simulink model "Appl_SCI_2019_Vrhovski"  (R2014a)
settings: Solver=ode45  StartTime=0.0  StopTime=1000  MaxStep=0.01  RelTol=1e-3
undefined symbols (not defined in the file): deg, H, kg, m, M, mm, N, rad, s, X, Y, Z
libraries: sm_lib x389, nesl_utility x69, simulink x7
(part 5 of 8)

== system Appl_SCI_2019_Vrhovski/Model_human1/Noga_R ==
  koljeno : Subsystem
  natkoljenica : Subsystem
  potkoljenica : Subsystem
  skocni_zglob_R : Subsystem
  skocni_zglob_R Joint : sm_lib/Joints/Universal Joint  SenseConstraintForce=off  SenseConstraintForceX=off  SenseConstraintForceY=off  SenseConstraintForceZ=off  SenseConstraintTorque=off  SenseConstraintTorqueX=off  SenseConstraintTorqueY=off  SenseConstraintTorqueZ=off  SenseTotalForce=off  SenseTotalForceX=off  SenseTotalForceY=off  SenseTotalForceZ=off  SenseTotalTorque=off  SenseTotalTorqueX=off  SenseTotalTorqueY=off  SenseTotalTorqueZ=off  CompositeWrenchDir=FollowerOnBase  CompositeWrenchFrame=BaseFrame  RxEquilibriumPosition=0  RxEquilibriumPositionUnits=deg  RxSpringStiffness=0  RxSpringStiffnessUnits=N*m/deg  RxDampingCoefficient=0  RxDampingCoefficientUnits=N*m/(deg/s)  RxTorqueActuationMode=ComputedTorque  RxMotionActuationMode=InputMotion  RxSensePosition=off  RxSenseVelocity=off  RxSenseAcceleration=off  RxSenseTorqueForce=off  RxPositionTargetValue=-0.08  RxPositionTargetValueUnits=rad  RxPositionTargetSpecify=on  RxPositionTargetPriority=High  RxVelocityTargetValue=0  RxVelocityTargetValueUnits=deg/s  RxVelocityTargetSpecify=off  RxVelocityTargetPriority=High  RyEquilibriumPosition=0  RyEquilibriumPositionUnits=deg  RySpringStiffness=0  RySpringStiffnessUnits=N*m/deg  RyDampingCoefficient=0  RyDampingCoefficientUnits=N*m/(deg/s)  RyTorqueActuationMode=ComputedTorque  RyMotionActuationMode=InputMotion  RySensePosition=off  RySenseVelocity=off  RySenseAcceleration=off  RySenseTorqueForce=off  RyPositionTargetValue=0  RyPositionTargetValueUnits=deg  RyPositionTargetSpecify=off  RyPositionTargetPriority=High  RyVelocityTargetValue=0  RyVelocityTargetValueUnits=deg/s  RyVelocityTargetSpecify=off  RyVelocityTargetPriority=High  BlockFunction=simmechanics.library.joints.universal_joint
  B : PMIOPort  Port=1  Side=Left
  F : PMIOPort  Port=2  Side=Right
  Nagib_skocnog : PMIOPort  Port=3  Side=Left
  RL1 : PMIOPort  Port=4  Side=Right
  RL2 : PMIOPort  Port=5  Side=Right
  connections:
  F/RConn1 -- natkoljenica/RConn1
  B/RConn1 -- skocni_zglob_R/LConn1
  koljeno/LConn1 -- potkoljenica/RConn1
  potkoljenica/LConn1 -- skocni_zglob_R Joint/RConn1
  skocni_zglob_R Joint/LConn1 -- RL1/RConn1 -- skocni_zglob_R/RConn1
  koljeno/RConn1 -- RL2/RConn1 -- natkoljenica/LConn1
  Nagib_skocnog/RConn1 -- skocni_zglob_R Joint/LConn3

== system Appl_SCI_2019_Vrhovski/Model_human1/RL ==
  L1 : Subsystem
  L2 : Subsystem
  L3 : Subsystem
  B : PMIOPort  Port=1  Side=Left
  FL1 : PMIOPort  Port=2  Side=Left
  FL2 : PMIOPort  Port=3  Side=Left
  FL3 : PMIOPort  Port=4  Side=Left
  Lxyz1 : Outport
  Lxyz2 : Outport  Port=2
  Lxyz3 : Outport  Port=3
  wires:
  L2/1(xyz) -> Lxyz2/1
  L3/1(xyz) -> Lxyz3/1
  L1/1(xyz) -> Lxyz1/1
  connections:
  FL2/RConn1 -- L2/LConn2
  L1/LConn2 -- FL1/RConn1
  L3/LConn2 -- FL3/RConn1
  B/RConn1 -- L1/LConn1 -- L3/LConn1 -- L2/LConn1

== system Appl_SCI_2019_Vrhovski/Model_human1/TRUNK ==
  T1 : Subsystem
  T2 : Subsystem
  T3 : Subsystem
  B : PMIOPort  Port=1  Side=Left
  FT1 : PMIOPort  Port=2  Side=Left
  FT2 : PMIOPort  Port=3  Side=Left
  FT3 : PMIOPort  Port=4  Side=Left
  Txyz1 : Outport
  Txyz2 : Outport  Port=2
  Txyz3 : Outport  Port=3
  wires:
  T1/1(xyz) -> Txyz1/1
  T3/1(xyz) -> Txyz3/1
  T2/1(xyz) -> Txyz2/1
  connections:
  T2/LConn1 -- T3/LConn1 -- T1/LConn1 -- B/RConn1
  T3/LConn2 -- FT3/RConn1
  T1/LConn2 -- FT1/RConn1
  FT2/RConn1 -- T2/LConn2

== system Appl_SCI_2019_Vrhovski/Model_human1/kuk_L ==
  Revolute Joint1 : sm_lib/Joints/Revolute Joint  SenseConstraintForce=off  SenseConstraintForceX=off  SenseConstraintForceY=off  SenseConstraintForceZ=off  SenseConstraintTorque=off  SenseConstraintTorqueX=off  SenseConstraintTorqueY=off  SenseConstraintTorqueZ=off  SenseTotalForce=off  SenseTotalForceX=off  SenseTotalForceY=off  SenseTotalForceZ=off  SenseTotalTorque=off  SenseTotalTorqueX=off  SenseTotalTorqueY=off  SenseTotalTorqueZ=off  CompositeWrenchDir=FollowerOnBase  CompositeWrenchFrame=BaseFrame  EquilibriumPosition=0  EquilibriumPositionUnits=deg  SpringStiffness=0  SpringStiffnessUnits=N*m/deg  DampingCoefficient=0  DampingCoefficientUnits=N*m/(deg/s)  TorqueActuationMode=NoTorque  MotionActuationMode=ComputedMotion  SensePosition=off  SenseVelocity=off  SenseAcceleration=off  SenseTorqueForce=off  PositionTargetValue=0  PositionTargetValueUnits=deg  PositionTargetSpecify=off  PositionTargetPriority=High  VelocityTargetValue=0  VelocityTargetValueUnits=deg/s  VelocityTargetSpecify=off  VelocityTargetPriority=High  BlockFunction=simmechanics.library.joints.revolute_joint
  Transform : sm_lib/Frames and Transforms/Rigid Transform  TranslationMethod=None  TranslationLengthUnit=mm  TranslationStandardAxis=+Z  TranslationStandardOffset=0  TranslationCartesianOffset=[-2.2026824808563106e-13 549.99999999999943 3.4106051316484809e-13]  TranslationROffset=0  TranslationROffsetUnits=m  TranslationZOffset=0  TranslationZOffsetUnits=m  TranslationThetaOffset=0  TranslationThetaOffsetUnits=deg  RotationMethod=StandardAxis  RotationAngleUnits=rad  RotationStandardAxis=+X  RotationAngle=pi/2  RotationArbitraryAxis=[0.57735026918962595 -0.57735026918962618 0.57735026918962518]  FollAlignAxisA=+X  BaseAlignAxisA=+Y  FollAlignAxisB=+Y  BaseAlignAxisB=+Z  BlockFunction=simmechanics.library.frames_transforms.rigid_transform
  Transform1 : sm_lib/Frames and Transforms/Rigid Transform  TranslationMethod=None  TranslationLengthUnit=mm  TranslationStandardAxis=+Z  TranslationStandardOffset=0  TranslationCartesianOffset=[-2.2026824808563106e-13 549.99999999999943 3.4106051316484809e-13]  TranslationROffset=0  TranslationROffsetUnits=m  TranslationZOffset=0  TranslationZOffsetUnits=m  TranslationThetaOffset=0  TranslationThetaOffsetUnits=deg  RotationMethod=StandardAxis  RotationAngleUnits=rad  RotationStandardAxis=-X  RotationAngle=pi/2  RotationArbitraryAxis=[0.57735026918962595 -0.57735026918962618 0.57735026918962518]  FollAlignAxisA=+X  BaseAlignAxisA=+Y  FollAlignAxisB=+Y  BaseAlignAxisB=+Z  BlockFunction=simmechanics.library.frames_transforms.rigid_transform
  kuk : Subsystem
  kuk_in : PMIOPort  Port=1  Side=Left
  kuk_out : PMIOPort  Port=2  Side=Right
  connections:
  Transform1/RConn1 -- kuk_out/RConn1
  Transform1/LConn1 -- Revolute Joint1/RConn1
  Transform/RConn1 -- Revolute Joint1/LConn1
  Transform/LConn1 -- kuk/RConn1
  kuk_in/RConn1 -- kuk/LConn1

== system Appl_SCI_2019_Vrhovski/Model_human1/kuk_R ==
  Revolute Joint1 : sm_lib/Joints/Revolute Joint  SenseConstraintForce=off  SenseConstraintForceX=off  SenseConstraintForceY=off  SenseConstraintForceZ=off  SenseConstraintTorque=off  SenseConstraintTorqueX=off  SenseConstraintTorqueY=off  SenseConstraintTorqueZ=off  SenseTotalForce=off  SenseTotalForceX=off  SenseTotalForceY=off  SenseTotalForceZ=off  SenseTotalTorque=off  SenseTotalTorqueX=off  SenseTotalTorqueY=off  SenseTotalTorqueZ=off  CompositeWrenchDir=FollowerOnBase  CompositeWrenchFrame=BaseFrame  EquilibriumPosition=0  EquilibriumPositionUnits=deg  SpringStiffness=0  SpringStiffnessUnits=N*m/deg  DampingCoefficient=0  DampingCoefficientUnits=N*m/(deg/s)  TorqueActuationMode=NoTorque  MotionActuationMode=ComputedMotion  SensePosition=off  SenseVelocity=off  SenseAcceleration=off  SenseTorqueForce=off  PositionTargetValue=0  PositionTargetValueUnits=deg  PositionTargetSpecify=off  PositionTargetPriority=High  VelocityTargetValue=0  VelocityTargetValueUnits=deg/s  VelocityTargetSpecify=off  VelocityTargetPriority=High  BlockFunction=simmechanics.library.joints.revolute_joint
  Transform : sm_lib/Frames and Transforms/Rigid Transform  TranslationMethod=None  TranslationLengthUnit=mm  TranslationStandardAxis=+Z  TranslationStandardOffset=0  TranslationCartesianOffset=[-2.2026824808563106e-13 549.99999999999943 3.4106051316484809e-13]  TranslationROffset=0  TranslationROffsetUnits=m  TranslationZOffset=0  TranslationZOffsetUnits=m  TranslationThetaOffset=0  TranslationThetaOffsetUnits=deg  RotationMethod=StandardAxis  RotationAngleUnits=rad  RotationStandardAxis=+X  RotationAngle=pi/2  RotationArbitraryAxis=[0.57735026918962595 -0.57735026918962618 0.57735026918962518]  FollAlignAxisA=+X  BaseAlignAxisA=+Y  FollAlignAxisB=+Y  BaseAlignAxisB=+Z  BlockFunction=simmechanics.library.frames_transforms.rigid_transform
  Transform1 : sm_lib/Frames and Transforms/Rigid Transform  TranslationMethod=None  TranslationLengthUnit=mm  TranslationStandardAxis=+Z  TranslationStandardOffset=0  TranslationCartesianOffset=[-2.2026824808563106e-13 549.99999999999943 3.4106051316484809e-13]  TranslationROffset=0  TranslationROffsetUnits=m  TranslationZOffset=0  TranslationZOffsetUnits=m  TranslationThetaOffset=0  TranslationThetaOffsetUnits=deg  RotationMethod=StandardAxis  RotationAngleUnits=rad  RotationStandardAxis=-X  RotationAngle=pi/2  RotationArbitraryAxis=[0.57735026918962595 -0.57735026918962618 0.57735026918962518]  FollAlignAxisA=+X  BaseAlignAxisA=+Y  FollAlignAxisB=+Y  BaseAlignAxisB=+Z  BlockFunction=simmechanics.library.frames_transforms.rigid_transform
  kuk : Subsystem
  kuk_in : PMIOPort  Port=1  Side=Left
  kuk_out : PMIOPort  Port=2  Side=Right
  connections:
  kuk_in/RConn1 -- kuk/LConn1
  Transform/LConn1 -- kuk/RConn1
  Transform/RConn1 -- Revolute Joint1/LConn1
  Transform1/LConn1 -- Revolute Joint1/RConn1
  Transform1/RConn1 -- kuk_out/RConn1

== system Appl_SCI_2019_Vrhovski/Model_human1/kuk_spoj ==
  ReferenceFrame : sm_lib/Frames and Transforms/Reference Frame  BlockFunction=simmechanics.library.frames_transforms.reference_frame
  Solid : sm_lib/Body Elements/Solid  InertiaType=Custom  Mass=0.1117*M  MassUnits=kg  CenterOfMass=[0 0 0]  CenterOfMassUnits=mm  MomentsOfInertia=[9638.0119049841542 90952.357607822152 82817.580647608978]  MomentsOfInertiaUnits=kg*mm^2  ProductsOfInertia=[101.02531458452592 0 0]  ProductsOfInertiaUnits=kg*mm^2  DensityBased=on  Density=1000  DensityUnits=kg/(m^3)  GraphicType=FromGeometry  MarkerShape=Sphere  MarkerSize=10  MarkerSizeUnits=m  GraphicVisPropType=SimpleVisualProperties  GraphicDiffuseColor=[0.792156862745098 0.81960784313725488 0.93333333333333335]  GraphicSpecularColor=[0.5 0.5 0.5 1.0]  GraphicAmbientColor=[0.15 0.15 0.15 1.0]  GraphicEmissiveColor=[0.0 0.0 0.0 1.0]  GraphicShininess=75  GraphicOpacity=1  GeometryShape=Ellipsoid  RectangleSize=[1 1]  RectangleSizeUnits=m  BrickDimensions=[330 50 50]  BrickDimensionUnits=mm  CylinderRadius=1  CylinderRadiusUnits=m  CylinderLength=1  CylinderLengthUnits=m  SphereRadius=1  SphereRadiusUnits=m  EllipsoidRadii=[175 50 0.05*H*5]  EllipsoidRadiiUnits=mm  ExtrusionCrossSection=[1 1; -1 1; -1 -1; 1 -1]  ExtrusionCrossSectionUnits=m  ExtrusionLength=1  ExtrusionLengthUnits=m  PolygonNumSides=3  PolygonOuterRadius=1  PolygonOuterRadiusUnits=m  ExtGeomFileType=STL  ExtGeomFileName=Spojnica_Default_sldprt.STL  ExtGeomFileUnits=mm  RevolutionCrossSection=[1 1; 1 -1; 2 -1; 2 1]  RevolutionCrossSectionUnits=m  RevolutionExtent=Full  RevolutionAngle=180  RevolutionAngleUnits=deg  BlockFunction=simmechanics.library.body_elements.solid
  Transform1 : sm_lib/Frames and Transforms/Rigid Transform  TranslationMethod=Cartesian  TranslationLengthUnit=mm  TranslationStandardAxis=+Z  TranslationStandardOffset=0  TranslationCartesianOffset=[132.5 0 0]  TranslationROffset=0  TranslationROffsetUnits=m  TranslationZOffset=0  TranslationZOffsetUnits=m  TranslationThetaOffset=0  TranslationThetaOffsetUnits=deg  RotationMethod=None  RotationAngleUnits=rad  RotationStandardAxis=+X  RotationAngle=pi  RotationArbitraryAxis=[0 0 0]  FollAlignAxisA=+X  BaseAlignAxisA=+Y  FollAlignAxisB=+Y  BaseAlignAxisB=+Z  BlockFunction=simmechanics.library.frames_transforms.rigid_transform
  Transform2 : sm_lib/Frames and Transforms/Rigid Transform  TranslationMethod=Cartesian  TranslationLengthUnit=mm  TranslationStandardAxis=+Z  TranslationStandardOffset=0  TranslationCartesianOffset=[-132.5 0 0]  TranslationROffset=0  TranslationROffsetUnits=m  TranslationZOffset=0  TranslationZOffsetUnits=m  TranslationThetaOffset=0  TranslationThetaOffsetUnits=deg  RotationMethod=None  RotationAngleUnits=rad  RotationStandardAxis=+X  RotationAngle=pi  RotationArbitraryAxis=[0 0 0]  FollAlignAxisA=+X  BaseAlignAxisA=+Y  FollAlignAxisB=+Y  BaseAlignAxisB=+Z  BlockFunction=simmechanics.library.frames_transforms.rigid_transform
  Transform3 : sm_lib/Frames and Transforms/Rigid Transform  TranslationMethod=None  TranslationLengthUnit=mm  TranslationStandardAxis=+Z  TranslationStandardOffset=0  TranslationCartesianOffset=[0 -0 -0]  TranslationROffset=0  TranslationROffsetUnits=m  TranslationZOffset=0  TranslationZOffsetUnits=m  TranslationThetaOffset=0  TranslationThetaOffsetUnits=deg  RotationMethod=None  RotationAngleUnits=rad  RotationStandardAxis=+X  RotationAngle=pi  RotationArbitraryAxis=[0 0 0]  FollAlignAxisA=+X  BaseAlignAxisA=+Y  FollAlignAxisB=+Y  BaseAlignAxisB=+Z  BlockFunction=simmechanics.library.frames_transforms.rigid_transform
  BL : PMIOPort  Port=1  Side=Right
  BR : PMIOPort  Port=2  Side=Right
  F : PMIOPort  Port=3  Side=Left
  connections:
  ReferenceFrame/RConn1 -- Transform3/LConn1 -- Solid/RConn1 -- Transform1/LConn1 -- Transform2/LConn1
  Transform1/RConn1 -- BR/RConn1
  Transform2/RConn1 -- BL/RConn1
  Transform3/RConn1 -- F/RConn1

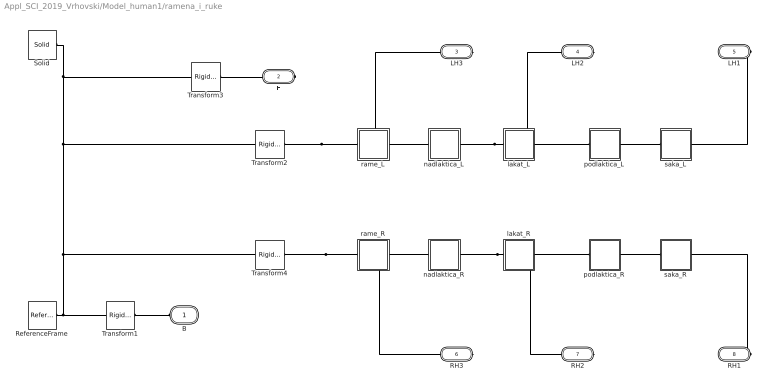
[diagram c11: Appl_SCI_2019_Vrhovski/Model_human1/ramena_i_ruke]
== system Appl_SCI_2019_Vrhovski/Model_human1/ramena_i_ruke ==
  ReferenceFrame : sm_lib/Frames and Transforms/Reference Frame  BlockFunction=simmechanics.library.frames_transforms.reference_frame
  Solid : sm_lib/Body Elements/Solid  InertiaType=Custom  Mass=0  MassUnits=kg  CenterOfMass=[0 0 0]  CenterOfMassUnits=mm  MomentsOfInertia=[9638.0119049841542 90952.357607822152 82817.580647608978]  MomentsOfInertiaUnits=kg*mm^2  ProductsOfInertia=[101.02531458452592 0 0]  ProductsOfInertiaUnits=kg*mm^2  DensityBased=on  Density=1000  DensityUnits=kg/(m^3)  GraphicType=FromGeometry  MarkerShape=Sphere  MarkerSize=10  MarkerSizeUnits=m  GraphicVisPropType=SimpleVisualProperties  GraphicDiffuseColor=[0.792156862745098 0.81960784313725488 0.93333333333333335]  GraphicSpecularColor=[0.5 0.5 0.5 1.0]  GraphicAmbientColor=[0.15 0.15 0.15 1.0]  GraphicEmissiveColor=[0.0 0.0 0.0 1.0]  GraphicShininess=75  GraphicOpacity=1  GeometryShape=Ellipsoid  RectangleSize=[1 1]  RectangleSizeUnits=m  BrickDimensions=[460 50 50]  BrickDimensionUnits=mm  CylinderRadius=1  CylinderRadiusUnits=m  CylinderLength=1  CylinderLengthUnits=m  SphereRadius=1  SphereRadiusUnits=m  EllipsoidRadii=[230 25 25]  EllipsoidRadiiUnits=mm  ExtrusionCrossSection=[1 1; -1 1; -1 -1; 1 -1]  ExtrusionCrossSectionUnits=m  ExtrusionLength=1  ExtrusionLengthUnits=m  PolygonNumSides=3  PolygonOuterRadius=1  PolygonOuterRadiusUnits=m  ExtGeomFileType=STL  ExtGeomFileName=Spojnica_Default_sldprt.STL  ExtGeomFileUnits=mm  RevolutionCrossSection=[1 1; 1 -1; 2 -1; 2 1]  RevolutionCrossSectionUnits=m  RevolutionExtent=Full  RevolutionAngle=180  RevolutionAngleUnits=deg  BlockFunction=simmechanics.library.body_elements.solid
  Transform1 : sm_lib/Frames and Transforms/Rigid Transform  TranslationMethod=StandardAxis  TranslationLengthUnit=mm  TranslationStandardAxis=+Z  TranslationStandardOffset=225  TranslationCartesianOffset=[150 0 0]  TranslationROffset=0  TranslationROffsetUnits=m  TranslationZOffset=0  TranslationZOffsetUnits=m  TranslationThetaOffset=0  TranslationThetaOffsetUnits=deg  RotationMethod=None  RotationAngleUnits=rad  RotationStandardAxis=+X  RotationAngle=pi  RotationArbitraryAxis=[0 0 0]  FollAlignAxisA=+X  BaseAlignAxisA=+Y  FollAlignAxisB=+Y  BaseAlignAxisB=+Z  BlockFunction=simmechanics.library.frames_transforms.rigid_transform
  Transform2 : sm_lib/Frames and Transforms/Rigid Transform  TranslationMethod=Cartesian  TranslationLengthUnit=mm  TranslationStandardAxis=+Z  TranslationStandardOffset=150  TranslationCartesianOffset=[200 0 -0]  TranslationROffset=0  TranslationROffsetUnits=m  TranslationZOffset=0  TranslationZOffsetUnits=m  TranslationThetaOffset=0  TranslationThetaOffsetUnits=deg  RotationMethod=StandardAxis  RotationAngleUnits=rad  RotationStandardAxis=+X  RotationAngle=pi  RotationArbitraryAxis=[0 0 0]  FollAlignAxisA=+X  BaseAlignAxisA=+Y  FollAlignAxisB=+Y  BaseAlignAxisB=+Z  BlockFunction=simmechanics.library.frames_transforms.rigid_transform
  Transform3 : sm_lib/Frames and Transforms/Rigid Transform  TranslationMethod=StandardAxis  TranslationLengthUnit=mm  TranslationStandardAxis=+Z  TranslationStandardOffset=150  TranslationCartesianOffset=[0 -0 -0]  TranslationROffset=0  TranslationROffsetUnits=m  TranslationZOffset=0  TranslationZOffsetUnits=m  TranslationThetaOffset=0  TranslationThetaOffsetUnits=deg  RotationMethod=None  RotationAngleUnits=rad  RotationStandardAxis=+X  RotationAngle=pi  RotationArbitraryAxis=[0 0 0]  FollAlignAxisA=+X  BaseAlignAxisA=+Y  FollAlignAxisB=+Y  BaseAlignAxisB=+Z  BlockFunction=simmechanics.library.frames_transforms.rigid_transform
  Transform4 : sm_lib/Frames and Transforms/Rigid Transform  TranslationMethod=Cartesian  TranslationLengthUnit=mm  TranslationStandardAxis=+Z  TranslationStandardOffset=150  TranslationCartesianOffset=[-200 0 -0]  TranslationROffset=0  TranslationROffsetUnits=m  TranslationZOffset=0  TranslationZOffsetUnits=m  TranslationThetaOffset=0  TranslationThetaOffsetUnits=deg  RotationMethod=StandardAxis  RotationAngleUnits=rad  RotationStandardAxis=+X  RotationAngle=pi  RotationArbitraryAxis=[0 0 0]  FollAlignAxisA=+X  BaseAlignAxisA=+Y  FollAlignAxisB=+Y  BaseAlignAxisB=+Z  BlockFunction=simmechanics.library.frames_transforms.rigid_transform
  lakat_L : Subsystem
  lakat_R : Subsystem
  nadlaktica_L : Subsystem
  nadlaktica_R : Subsystem
  podlaktica_L : Subsystem
  podlaktica_R : Subsystem
  rame_L : Subsystem
  rame_R : Subsystem
  saka_L : Subsystem
  saka_R : Subsystem
  B : PMIOPort  Port=1  Side=Left
  F : PMIOPort  Port=2  Side=Right
  LH3 : PMIOPort  Port=3  Side=Right
  LH2 : PMIOPort  Port=4  Side=Right
  LH1 : PMIOPort  Port=5  Side=Right
  RH3 : PMIOPort  Port=6  Side=Right
  RH2 : PMIOPort  Port=7  Side=Right
  RH1 : PMIOPort  Port=8  Side=Right
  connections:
  ReferenceFrame/RConn1 -- Transform1/LConn1 -- Transform4/LConn1 -- Transform2/LConn1 -- Transform3/LConn1 -- Solid/RConn1
  Transform1/RConn1 -- B/RConn1
  Transform3/RConn1 -- F/RConn1
  Transform2/RConn1 -- LH3/RConn1 -- rame_L/LConn1
  lakat_L/LConn1 -- LH2/RConn1 -- nadlaktica_L/RConn1
  saka_L/LConn1 -- podlaktica_L/RConn1
  saka_R/LConn1 -- podlaktica_R/RConn1
  lakat_R/LConn1 -- RH2/RConn1 -- nadlaktica_R/RConn1
  Transform4/RConn1 -- RH3/RConn1 -- rame_R/LConn1
  rame_L/RConn1 -- nadlaktica_L/LConn1
  nadlaktica_R/LConn1 -- rame_R/RConn1
  lakat_L/RConn1 -- podlaktica_L/LConn1
  lakat_R/RConn1 -- podlaktica_R/LConn1
  LH1/RConn1 -- saka_L/RConn1
  RH1/RConn1 -- saka_R/RConn1

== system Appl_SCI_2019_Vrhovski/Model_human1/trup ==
  ReferenceFrame : sm_lib/Frames and Transforms/Reference Frame  BlockFunction=simmechanics.library.frames_transforms.reference_frame
  Solid : sm_lib/Body Elements/Solid  InertiaType=Custom  Mass=0.1633*M  MassUnits=kg  CenterOfMass=[0 0 0]  CenterOfMassUnits=mm  MomentsOfInertia=[2897.1863857204326 1.8962829928219973 2897.1862300567827]  MomentsOfInertiaUnits=kg*mm^2  ProductsOfInertia=[0 0 -0.00027890183916846033]  ProductsOfInertiaUnits=kg*mm^2  DensityBased=on  Density=1000  DensityUnits=kg/(m^3)  GraphicType=FromGeometry  MarkerShape=Sphere  MarkerSize=10  MarkerSizeUnits=m  GraphicVisPropType=SimpleVisualProperties  GraphicDiffuseColor=[0.792156862745098 0.81960784313725488 0.93333333333333335]  GraphicSpecularColor=[0.5 0.5 0.5 1.0]  GraphicAmbientColor=[0.15 0.15 0.15 1.0]  GraphicEmissiveColor=[0.0 0.0 0.0 1.0]  GraphicShininess=75  GraphicOpacity=1  GeometryShape=Ellipsoid  RectangleSize=[1 1]  RectangleSizeUnits=m  BrickDimensions=[1 1 1]  BrickDimensionUnits=m  CylinderRadius=2.5  CylinderRadiusUnits=cm  CylinderLength=22  CylinderLengthUnits=cm  SphereRadius=5  SphereRadiusUnits=cm  EllipsoidRadii=[150 50 0.107*H*5]  EllipsoidRadiiUnits=mm  ExtrusionCrossSection=[1 1; -1 1; -1 -1; 1 -1]  ExtrusionCrossSectionUnits=m  ExtrusionLength=1  ExtrusionLengthUnits=m  PolygonNumSides=3  PolygonOuterRadius=1  PolygonOuterRadiusUnits=m  ExtGeomFileType=STL  ExtGeomFileName=Pod_Default_sldprt.STL  ExtGeomFileUnits=mm  RevolutionCrossSection=[1 1; 1 -1; 2 -1; 2 1]  RevolutionCrossSectionUnits=m  RevolutionExtent=Full  RevolutionAngle=180  RevolutionAngleUnits=deg  BlockFunction=simmechanics.library.body_elements.solid
  Transform1 : sm_lib/Frames and Transforms/Rigid Transform  TranslationMethod=StandardAxis  TranslationLengthUnit=mm  TranslationStandardAxis=+Z  TranslationStandardOffset=0.107*H*5 +10  TranslationCartesianOffset=[1.3358203432289883e-12 650.00000000000045 -1.0913936421275139e-11]  TranslationROffset=0  TranslationROffsetUnits=m  TranslationZOffset=0  TranslationZOffsetUnits=m  TranslationThetaOffset=0  TranslationThetaOffsetUnits=deg  RotationMethod=None  RotationAngleUnits=rad  RotationStandardAxis=+Z  RotationAngle=0  RotationArbitraryAxis=[0 0 0]  FollAlignAxisA=+X  BaseAlignAxisA=+Y  FollAlignAxisB=+Y  BaseAlignAxisB=+Z  BlockFunction=simmechanics.library.frames_transforms.rigid_transform
  Transform3 : sm_lib/Frames and Transforms/Rigid Transform  TranslationMethod=StandardAxis  TranslationLengthUnit=mm  TranslationStandardAxis=-Z  TranslationStandardOffset=0.107*H*5 +10  TranslationCartesianOffset=[-2.2026824808563106e-13 549.99999999999943 3.4106051316484809e-13]  TranslationROffset=0  TranslationROffsetUnits=m  TranslationZOffset=0  TranslationZOffsetUnits=m  TranslationThetaOffset=0  TranslationThetaOffsetUnits=deg  RotationMethod=None  RotationAngleUnits=rad  RotationStandardAxis=+Z  RotationAngle=2.0943951023931962  RotationArbitraryAxis=[0.57735026918962595 -0.57735026918962618 0.57735026918962518]  FollAlignAxisA=+X  BaseAlignAxisA=+Y  FollAlignAxisB=+Y  BaseAlignAxisB=+Z  BlockFunction=simmechanics.library.frames_transforms.rigid_transform
  F : PMIOPort  Port=1  Side=Right
  B : PMIOPort  Port=2  Side=Left
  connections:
  Transform1/LConn1 -- ReferenceFrame/RConn1 -- Solid/RConn1 -- Transform3/LConn1
  Transform1/RConn1 -- F/RConn1
  Transform3/RConn1 -- B/RConn1

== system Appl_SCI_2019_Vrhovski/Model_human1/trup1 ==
  ReferenceFrame : sm_lib/Frames and Transforms/Reference Frame  BlockFunction=simmechanics.library.frames_transforms.reference_frame
  Solid : sm_lib/Body Elements/Solid  InertiaType=Custom  Mass=0.17275*M  MassUnits=kg  CenterOfMass=[0 0 0]  CenterOfMassUnits=mm  MomentsOfInertia=[2897.1863857204326 1.8962829928219973 2897.1862300567827]  MomentsOfInertiaUnits=kg*mm^2  ProductsOfInertia=[0 0 -0.00027890183916846033]  ProductsOfInertiaUnits=kg*mm^2  DensityBased=on  Density=1000  DensityUnits=kg/(m^3)  GraphicType=FromGeometry  MarkerShape=Sphere  MarkerSize=10  MarkerSizeUnits=m  GraphicVisPropType=SimpleVisualProperties  GraphicDiffuseColor=[0.792156862745098 0.81960784313725488 0.93333333333333335]  GraphicSpecularColor=[0.5 0.5 0.5 1.0]  GraphicAmbientColor=[0.15 0.15 0.15 1.0]  GraphicEmissiveColor=[0.0 0.0 0.0 1.0]  GraphicShininess=75  GraphicOpacity=1  GeometryShape=Ellipsoid  RectangleSize=[1 1]  RectangleSizeUnits=m  BrickDimensions=[1 1 1]  BrickDimensionUnits=m  CylinderRadius=2.5  CylinderRadiusUnits=cm  CylinderLength=22  CylinderLengthUnits=cm  SphereRadius=5  SphereRadiusUnits=cm  EllipsoidRadii=[150 50 0.181*H*5]  EllipsoidRadiiUnits=mm  ExtrusionCrossSection=[1 1; -1 1; -1 -1; 1 -1]  ExtrusionCrossSectionUnits=m  ExtrusionLength=1  ExtrusionLengthUnits=m  PolygonNumSides=3  PolygonOuterRadius=1  PolygonOuterRadiusUnits=m  ExtGeomFileType=STL  ExtGeomFileName=Pod_Default_sldprt.STL  ExtGeomFileUnits=mm  RevolutionCrossSection=[1 1; 1 -1; 2 -1; 2 1]  RevolutionCrossSectionUnits=m  RevolutionExtent=Full  RevolutionAngle=180  RevolutionAngleUnits=deg  BlockFunction=simmechanics.library.body_elements.solid
  Transform1 : sm_lib/Frames and Transforms/Rigid Transform  TranslationMethod=StandardAxis  TranslationLengthUnit=mm  TranslationStandardAxis=+Z  TranslationStandardOffset=0.181*H*5+10  TranslationCartesianOffset=[1.3358203432289883e-12 650.00000000000045 -1.0913936421275139e-11]  TranslationROffset=0  TranslationROffsetUnits=m  TranslationZOffset=0  TranslationZOffsetUnits=m  TranslationThetaOffset=0  TranslationThetaOffsetUnits=deg  RotationMethod=None  RotationAngleUnits=rad  RotationStandardAxis=+Z  RotationAngle=0  RotationArbitraryAxis=[0 0 0]  FollAlignAxisA=+X  BaseAlignAxisA=+Y  FollAlignAxisB=+Y  BaseAlignAxisB=+Z  BlockFunction=simmechanics.library.frames_transforms.rigid_transform
  Transform3 : sm_lib/Frames and Transforms/Rigid Transform  TranslationMethod=StandardAxis  TranslationLengthUnit=mm  TranslationStandardAxis=-Z  TranslationStandardOffset=0.181*H*5+10  TranslationCartesianOffset=[-2.2026824808563106e-13 549.99999999999943 3.4106051316484809e-13]  TranslationROffset=0  TranslationROffsetUnits=m  TranslationZOffset=0  TranslationZOffsetUnits=m  TranslationThetaOffset=0  TranslationThetaOffsetUnits=deg  RotationMethod=None  RotationAngleUnits=rad  RotationStandardAxis=+Z  RotationAngle=2.0943951023931962  RotationArbitraryAxis=[0.57735026918962595 -0.57735026918962618 0.57735026918962518]  FollAlignAxisA=+X  BaseAlignAxisA=+Y  FollAlignAxisB=+Y  BaseAlignAxisB=+Z  BlockFunction=simmechanics.library.frames_transforms.rigid_transform
  F : PMIOPort  Port=1  Side=Right
  B : PMIOPort  Port=2  Side=Left
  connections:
  Transform3/RConn1 -- B/RConn1
  Transform1/RConn1 -- F/RConn1
  Transform3/LConn1 -- Solid/RConn1 -- ReferenceFrame/RConn1 -- Transform1/LConn1

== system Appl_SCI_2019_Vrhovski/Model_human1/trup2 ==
  ReferenceFrame : sm_lib/Frames and Transforms/Reference Frame  BlockFunction=simmechanics.library.frames_transforms.reference_frame
  Solid : sm_lib/Body Elements/Solid  InertiaType=Custom  Mass=0  MassUnits=kg  CenterOfMass=[0 0 0]  CenterOfMassUnits=mm  MomentsOfInertia=[2897.1863857204326 1.8962829928219973 2897.1862300567827]  MomentsOfInertiaUnits=kg*mm^2  ProductsOfInertia=[0 0 -0.00027890183916846033]  ProductsOfInertiaUnits=kg*mm^2  DensityBased=on  Density=1000  DensityUnits=kg/(m^3)  GraphicType=FromGeometry  MarkerShape=Sphere  MarkerSize=10  MarkerSizeUnits=m  GraphicVisPropType=SimpleVisualProperties  GraphicDiffuseColor=[0.792156862745098 0.81960784313725488 0.93333333333333335]  GraphicSpecularColor=[0.5 0.5 0.5 1.0]  GraphicAmbientColor=[0.15 0.15 0.15 1.0]  GraphicEmissiveColor=[0.0 0.0 0.0 1.0]  GraphicShininess=75  GraphicOpacity=1  GeometryShape=Ellipsoid  RectangleSize=[1 1]  RectangleSizeUnits=m  BrickDimensions=[1 1 1]  BrickDimensionUnits=m  CylinderRadius=2.5  CylinderRadiusUnits=cm  CylinderLength=22  CylinderLengthUnits=mm  SphereRadius=5  SphereRadiusUnits=cm  EllipsoidRadii=[30 30 30]  EllipsoidRadiiUnits=mm  ExtrusionCrossSection=[1 1; -1 1; -1 -1; 1 -1]  ExtrusionCrossSectionUnits=m  ExtrusionLength=1  ExtrusionLengthUnits=m  PolygonNumSides=3  PolygonOuterRadius=1  PolygonOuterRadiusUnits=m  ExtGeomFileType=STL  ExtGeomFileName=Pod_Default_sldprt.STL  ExtGeomFileUnits=mm  RevolutionCrossSection=[1 1; 1 -1; 2 -1; 2 1]  RevolutionCrossSectionUnits=m  RevolutionExtent=Full  RevolutionAngle=180  RevolutionAngleUnits=deg  BlockFunction=simmechanics.library.body_elements.solid
  Transform1 : sm_lib/Frames and Transforms/Rigid Transform  TranslationMethod=StandardAxis  TranslationLengthUnit=mm  TranslationStandardAxis=+Z  TranslationStandardOffset=25  TranslationCartesianOffset=[1.3358203432289883e-12 650.00000000000045 -1.0913936421275139e-11]  TranslationROffset=0  TranslationROffsetUnits=m  TranslationZOffset=0  TranslationZOffsetUnits=m  TranslationThetaOffset=0  TranslationThetaOffsetUnits=deg  RotationMethod=None  RotationAngleUnits=rad  RotationStandardAxis=+Z  RotationAngle=0  RotationArbitraryAxis=[0 0 0]  FollAlignAxisA=+X  BaseAlignAxisA=+Y  FollAlignAxisB=+Y  BaseAlignAxisB=+Z  BlockFunction=simmechanics.library.frames_transforms.rigid_transform
  Transform3 : sm_lib/Frames and Transforms/Rigid Transform  TranslationMethod=StandardAxis  TranslationLengthUnit=mm  TranslationStandardAxis=-Z  TranslationStandardOffset=135  TranslationCartesianOffset=[-2.2026824808563106e-13 549.99999999999943 3.4106051316484809e-13]  TranslationROffset=0  TranslationROffsetUnits=m  TranslationZOffset=0  TranslationZOffsetUnits=m  TranslationThetaOffset=0  TranslationThetaOffsetUnits=deg  RotationMethod=None  RotationAngleUnits=rad  RotationStandardAxis=+Z  RotationAngle=2.0943951023931962  RotationArbitraryAxis=[0.57735026918962595 -0.57735026918962618 0.57735026918962518]  FollAlignAxisA=+X  BaseAlignAxisA=+Y  FollAlignAxisB=+Y  BaseAlignAxisB=+Z  BlockFunction=simmechanics.library.frames_transforms.rigid_transform
  F : PMIOPort  Port=1  Side=Right
  B : PMIOPort  Port=2  Side=Left
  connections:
  Transform1/LConn1 -- Solid/RConn1 -- ReferenceFrame/RConn1 -- Transform3/LConn1
  Transform1/RConn1 -- F/RConn1
  Transform3/RConn1 -- B/RConn1

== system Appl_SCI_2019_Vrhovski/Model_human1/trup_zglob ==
  ReferenceFrame : sm_lib/Frames and Transforms/Reference Frame  BlockFunction=simmechanics.library.frames_transforms.reference_frame
  Solid : sm_lib/Body Elements/Solid  InertiaType=Custom  Mass=0  MassUnits=kg  CenterOfMass=[0 0 0]  CenterOfMassUnits=mm  MomentsOfInertia=[2897.1863857204326 1.8962829928219973 2897.1862300567827]  MomentsOfInertiaUnits=kg*mm^2  ProductsOfInertia=[0 0 -0.00027890183916846033]  ProductsOfInertiaUnits=kg*mm^2  DensityBased=on  Density=1000  DensityUnits=kg/(m^3)  GraphicType=FromGeometry  MarkerShape=Sphere  MarkerSize=10  MarkerSizeUnits=m  GraphicVisPropType=SimpleVisualProperties  GraphicDiffuseColor=[0.792156862745098 0.81960784313725488 0.93333333333333335]  GraphicSpecularColor=[0.5 0.5 0.5 1.0]  GraphicAmbientColor=[0.15 0.15 0.15 1.0]  GraphicEmissiveColor=[0.0 0.0 0.0 1.0]  GraphicShininess=75  GraphicOpacity=1  GeometryShape=Sphere  RectangleSize=[1 1]  RectangleSizeUnits=m  BrickDimensions=[1 1 1]  BrickDimensionUnits=m  CylinderRadius=1  CylinderRadiusUnits=m  CylinderLength=1  CylinderLengthUnits=m  SphereRadius=3  SphereRadiusUnits=cm  EllipsoidRadii=[1 1 1]  EllipsoidRadiiUnits=m  ExtrusionCrossSection=[1 1; -1 1; -1 -1; 1 -1]  ExtrusionCrossSectionUnits=m  ExtrusionLength=1  ExtrusionLengthUnits=m  PolygonNumSides=3  PolygonOuterRadius=1  PolygonOuterRadiusUnits=m  ExtGeomFileType=STL  ExtGeomFileName=Pod_Default_sldprt.STL  ExtGeomFileUnits=mm  RevolutionCrossSection=[1 1; 1 -1; 2 -1; 2 1]  RevolutionCrossSectionUnits=m  RevolutionExtent=Full  RevolutionAngle=180  RevolutionAngleUnits=deg  BlockFunction=simmechanics.library.body_elements.solid
  Transform : sm_lib/Frames and Transforms/Rigid Transform  TranslationMethod=StandardAxis  TranslationLengthUnit=mm  TranslationStandardAxis=-Z  TranslationStandardOffset=0.05*H*5+25  TranslationCartesianOffset=[-2.2026824808563106e-13 549.99999999999943 3.4106051316484809e-13]  TranslationROffset=0  TranslationROffsetUnits=m  TranslationZOffset=0  TranslationZOffsetUnits=m  TranslationThetaOffset=0  TranslationThetaOffsetUnits=deg  RotationMethod=None  RotationAngleUnits=rad  RotationStandardAxis=+Z  RotationAngle=2.0943951023931962  RotationArbitraryAxis=[0.57735026918962595 -0.57735026918962618 0.57735026918962518]  FollAlignAxisA=+X  BaseAlignAxisA=+Y  FollAlignAxisB=+Y  BaseAlignAxisB=+Z  BlockFunction=simmechanics.library.frames_transforms.rigid_transform
  Transform1 : sm_lib/Frames and Transforms/Rigid Transform  TranslationMethod=None  TranslationLengthUnit=mm  TranslationStandardAxis=+Z  TranslationStandardOffset=0  TranslationCartesianOffset=[1.3358203432289883e-12 0 -1.0913936421275139e-11]  TranslationROffset=0  TranslationROffsetUnits=m  TranslationZOffset=0  TranslationZOffsetUnits=m  TranslationThetaOffset=0  TranslationThetaOffsetUnits=deg  RotationMethod=None  RotationAngleUnits=rad  RotationStandardAxis=+Z  RotationAngle=0  RotationArbitraryAxis=[0 0 0]  FollAlignAxisA=+X  BaseAlignAxisA=+Y  FollAlignAxisB=+Y  BaseAlignAxisB=+Z  BlockFunction=simmechanics.library.frames_transforms.rigid_transform
  F : PMIOPort  Port=1  Side=Right
  B : PMIOPort  Port=2  Side=Left
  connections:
  Transform1/RConn1 -- F/RConn1
  Transform/RConn1 -- B/RConn1
  Solid/RConn1 -- ReferenceFrame/RConn1 -- Transform1/LConn1 -- Transform/LConn1

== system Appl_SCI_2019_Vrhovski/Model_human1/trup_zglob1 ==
  ReferenceFrame : sm_lib/Frames and Transforms/Reference Frame  BlockFunction=simmechanics.library.frames_transforms.reference_frame
  Solid : sm_lib/Body Elements/Solid  InertiaType=Custom  Mass=0  MassUnits=kg  CenterOfMass=[0 0 0]  CenterOfMassUnits=mm  MomentsOfInertia=[2897.1863857204326 1.8962829928219973 2897.1862300567827]  MomentsOfInertiaUnits=kg*mm^2  ProductsOfInertia=[0 0 -0.00027890183916846033]  ProductsOfInertiaUnits=kg*mm^2  DensityBased=on  Density=1000  DensityUnits=kg/(m^3)  GraphicType=FromGeometry  MarkerShape=Sphere  MarkerSize=10  MarkerSizeUnits=m  GraphicVisPropType=SimpleVisualProperties  GraphicDiffuseColor=[0.792156862745098 0.81960784313725488 0.93333333333333335]  GraphicSpecularColor=[0.5 0.5 0.5 1.0]  GraphicAmbientColor=[0.15 0.15 0.15 1.0]  GraphicEmissiveColor=[0.0 0.0 0.0 1.0]  GraphicShininess=75  GraphicOpacity=1  GeometryShape=Sphere  RectangleSize=[1 1]  RectangleSizeUnits=m  BrickDimensions=[1 1 1]  BrickDimensionUnits=m  CylinderRadius=1  CylinderRadiusUnits=m  CylinderLength=1  CylinderLengthUnits=m  SphereRadius=2.5  SphereRadiusUnits=cm  EllipsoidRadii=[1 1 1]  EllipsoidRadiiUnits=m  ExtrusionCrossSection=[1 1; -1 1; -1 -1; 1 -1]  ExtrusionCrossSectionUnits=m  ExtrusionLength=1  ExtrusionLengthUnits=m  PolygonNumSides=3  PolygonOuterRadius=1  PolygonOuterRadiusUnits=m  ExtGeomFileType=STL  ExtGeomFileName=Pod_Default_sldprt.STL  ExtGeomFileUnits=mm  RevolutionCrossSection=[1 1; 1 -1; 2 -1; 2 1]  RevolutionCrossSectionUnits=m  RevolutionExtent=Full  RevolutionAngle=180  RevolutionAngleUnits=deg  BlockFunction=simmechanics.library.body_elements.solid
  Transform : sm_lib/Frames and Transforms/Rigid Transform  TranslationMethod=None  TranslationLengthUnit=mm  TranslationStandardAxis=+Z  TranslationStandardOffset=0  TranslationCartesianOffset=[-2.2026824808563106e-13 549.99999999999943 3.4106051316484809e-13]  TranslationROffset=0  TranslationROffsetUnits=m  TranslationZOffset=0  TranslationZOffsetUnits=m  TranslationThetaOffset=0  TranslationThetaOffsetUnits=deg  RotationMethod=None  RotationAngleUnits=rad  RotationStandardAxis=+Z  RotationAngle=2.0943951023931962  RotationArbitraryAxis=[0.57735026918962595 -0.57735026918962618 0.57735026918962518]  FollAlignAxisA=+X  BaseAlignAxisA=+Y  FollAlignAxisB=+Y  BaseAlignAxisB=+Z  BlockFunction=simmechanics.library.frames_transforms.rigid_transform
  Transform1 : sm_lib/Frames and Transforms/Rigid Transform  TranslationMethod=None  TranslationLengthUnit=mm  TranslationStandardAxis=+Z  TranslationStandardOffset=0  TranslationCartesianOffset=[1.3358203432289883e-12 0 -1.0913936421275139e-11]  TranslationROffset=0  TranslationROffsetUnits=m  TranslationZOffset=0  TranslationZOffsetUnits=m  TranslationThetaOffset=0  TranslationThetaOffsetUnits=deg  RotationMethod=None  RotationAngleUnits=rad  RotationStandardAxis=+Z  RotationAngle=0  RotationArbitraryAxis=[0 0 0]  FollAlignAxisA=+X  BaseAlignAxisA=+Y  FollAlignAxisB=+Y  BaseAlignAxisB=+Z  BlockFunction=simmechanics.library.frames_transforms.rigid_transform
  F : PMIOPort  Port=1  Side=Right
  B : PMIOPort  Port=2  Side=Left
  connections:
  Transform/LConn1 -- Transform1/LConn1 -- Solid/RConn1 -- ReferenceFrame/RConn1
  Transform/RConn1 -- B/RConn1
  Transform1/RConn1 -- F/RConn1

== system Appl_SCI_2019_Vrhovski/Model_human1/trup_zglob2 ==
  ReferenceFrame : sm_lib/Frames and Transforms/Reference Frame  BlockFunction=simmechanics.library.frames_transforms.reference_frame
  Solid : sm_lib/Body Elements/Solid  InertiaType=Custom  Mass=0  MassUnits=kg  CenterOfMass=[0 0 0]  CenterOfMassUnits=mm  MomentsOfInertia=[2897.1863857204326 1.8962829928219973 2897.1862300567827]  MomentsOfInertiaUnits=kg*mm^2  ProductsOfInertia=[0 0 -0.00027890183916846033]  ProductsOfInertiaUnits=kg*mm^2  DensityBased=on  Density=1000  DensityUnits=kg/(m^3)  GraphicType=FromGeometry  MarkerShape=Sphere  MarkerSize=10  MarkerSizeUnits=m  GraphicVisPropType=SimpleVisualProperties  GraphicDiffuseColor=[0.792156862745098 0.81960784313725488 0.93333333333333335]  GraphicSpecularColor=[0.5 0.5 0.5 1.0]  GraphicAmbientColor=[0.15 0.15 0.15 1.0]  GraphicEmissiveColor=[0.0 0.0 0.0 1.0]  GraphicShininess=75  GraphicOpacity=1  GeometryShape=Sphere  RectangleSize=[1 1]  RectangleSizeUnits=m  BrickDimensions=[1 1 1]  BrickDimensionUnits=m  CylinderRadius=1  CylinderRadiusUnits=m  CylinderLength=1  CylinderLengthUnits=m  SphereRadius=2.5  SphereRadiusUnits=cm  EllipsoidRadii=[1 1 1]  EllipsoidRadiiUnits=m  ExtrusionCrossSection=[1 1; -1 1; -1 -1; 1 -1]  ExtrusionCrossSectionUnits=m  ExtrusionLength=1  ExtrusionLengthUnits=m  PolygonNumSides=3  PolygonOuterRadius=1  PolygonOuterRadiusUnits=m  ExtGeomFileType=STL  ExtGeomFileName=Pod_Default_sldprt.STL  ExtGeomFileUnits=mm  RevolutionCrossSection=[1 1; 1 -1; 2 -1; 2 1]  RevolutionCrossSectionUnits=m  RevolutionExtent=Full  RevolutionAngle=180  RevolutionAngleUnits=deg  BlockFunction=simmechanics.library.body_elements.solid
  Transform : sm_lib/Frames and Transforms/Rigid Transform  TranslationMethod=None  TranslationLengthUnit=mm  TranslationStandardAxis=+Z  TranslationStandardOffset=0  TranslationCartesianOffset=[-2.2026824808563106e-13 549.99999999999943 3.4106051316484809e-13]  TranslationROffset=0  TranslationROffsetUnits=m  TranslationZOffset=0  TranslationZOffsetUnits=m  TranslationThetaOffset=0  TranslationThetaOffsetUnits=deg  RotationMethod=None  RotationAngleUnits=rad  RotationStandardAxis=+Z  RotationAngle=2.0943951023931962  RotationArbitraryAxis=[0.57735026918962595 -0.57735026918962618 0.57735026918962518]  FollAlignAxisA=+X  BaseAlignAxisA=+Y  FollAlignAxisB=+Y  BaseAlignAxisB=+Z  BlockFunction=simmechanics.library.frames_transforms.rigid_transform
  Transform1 : sm_lib/Frames and Transforms/Rigid Transform  TranslationMethod=None  TranslationLengthUnit=mm  TranslationStandardAxis=+Z  TranslationStandardOffset=0  TranslationCartesianOffset=[1.3358203432289883e-12 0 -1.0913936421275139e-11]  TranslationROffset=0  TranslationROffsetUnits=m  TranslationZOffset=0  TranslationZOffsetUnits=m  TranslationThetaOffset=0  TranslationThetaOffsetUnits=deg  RotationMethod=None  RotationAngleUnits=rad  RotationStandardAxis=+Z  RotationAngle=0  RotationArbitraryAxis=[0 0 0]  FollAlignAxisA=+X  BaseAlignAxisA=+Y  FollAlignAxisB=+Y  BaseAlignAxisB=+Z  BlockFunction=simmechanics.library.frames_transforms.rigid_transform
  F : PMIOPort  Port=1  Side=Right
  B : PMIOPort  Port=2  Side=Left
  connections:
  Transform1/RConn1 -- F/RConn1
  Transform/RConn1 -- B/RConn1
  ReferenceFrame/RConn1 -- Solid/RConn1 -- Transform1/LConn1 -- Transform/LConn1

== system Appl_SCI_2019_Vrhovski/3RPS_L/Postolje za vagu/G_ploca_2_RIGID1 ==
  ReferenceFrame : sm_lib/Frames and Transforms/Reference Frame  BlockFunction=simmechanics.library.frames_transforms.reference_frame
  Solid : sm_lib/Body Elements/Solid  InertiaType=Custom  Mass=5  MassUnits=kg  CenterOfMass=[-1.0925911726464245e-05 0 -4.4436244658035022]  CenterOfMassUnits=mm  MomentsOfInertia=[45540 79860 45540]  MomentsOfInertiaUnits=kg*mm^2  ProductsOfInertia=[0 -0.00010369999054466602 0]  ProductsOfInertiaUnits=kg*mm^2  DensityBased=on  Density=1000  DensityUnits=kg/(m^3)  GraphicType=FromGeometry  MarkerShape=Sphere  MarkerSize=10  MarkerSizeUnits=m  GraphicVisPropType=SimpleVisualProperties  GraphicDiffuseColor=[0.8 0.8 0.8]  GraphicSpecularColor=[0.5 0.5 0.5 1.0]  GraphicAmbientColor=[0.15 0.15 0.15 1.0]  GraphicEmissiveColor=[0.0 0.0 0.0 1.0]  GraphicShininess=75  GraphicOpacity=1  GeometryShape=Brick  RectangleSize=[1 1]  RectangleSizeUnits=m  BrickDimensions=[100 65 40]  BrickDimensionUnits=mm  CylinderRadius=120  CylinderRadiusUnits=mm  CylinderLength=20  CylinderLengthUnits=mm  SphereRadius=1  SphereRadiusUnits=m  EllipsoidRadii=[1 1 1]  EllipsoidRadiiUnits=m  ExtrusionCrossSection=[1 1; -1 1; -1 -1; 1 -1]  ExtrusionCrossSectionUnits=m  ExtrusionLength=1  ExtrusionLengthUnits=m  PolygonNumSides=3  PolygonOuterRadius=1  PolygonOuterRadiusUnits=m  ExtGeomFileType=STL  ExtGeomFileName=G_ploca_Default_sldprt.STL  ExtGeomFileUnits=mm  RevolutionCrossSection=[1 1; 1 -1; 2 -1; 2 1]  RevolutionCrossSectionUnits=m  RevolutionExtent=Full  RevolutionAngle=180  RevolutionAngleUnits=deg  BlockFunction=simmechanics.library.body_elements.solid
  Transform1 : sm_lib/Frames and Transforms/Rigid Transform  TranslationMethod=None  TranslationLengthUnit=mm  TranslationStandardAxis=-Z  TranslationStandardOffset=35.5  TranslationCartesianOffset="[-50.0000   86.6025         -10]"  TranslationROffset=0  TranslationROffsetUnits=m  TranslationZOffset=0  TranslationZOffsetUnits=m  TranslationThetaOffset=0  TranslationThetaOffsetUnits=deg  RotationMethod=ArbitraryAxis  RotationAngleUnits=rad  RotationStandardAxis=+Z  RotationAngle=0  RotationArbitraryAxis=[0 0 0]  FollAlignAxisA=+X  BaseAlignAxisA=+Y  FollAlignAxisB=+Y  BaseAlignAxisB=+Z  BlockFunction=simmechanics.library.frames_transforms.rigid_transform
  Transform3 : sm_lib/Frames and Transforms/Rigid Transform  TranslationMethod=None  TranslationLengthUnit=mm  TranslationStandardAxis=+Z  TranslationStandardOffset=35.5  TranslationCartesianOffset=[80.000000000002558 4.2632564145606011e-14 -32.999999999999048]  TranslationROffset=0  TranslationROffsetUnits=m  TranslationZOffset=0  TranslationZOffsetUnits=m  TranslationThetaOffset=0  TranslationThetaOffsetUnits=deg  RotationMethod=None  RotationAngleUnits=rad  RotationStandardAxis=+Z  RotationAngle=0  RotationArbitraryAxis=[0 0 0]  FollAlignAxisA=+X  BaseAlignAxisA=+Y  FollAlignAxisB=+Y  BaseAlignAxisB=+Z  BlockFunction=simmechanics.library.frames_transforms.rigid_transform
  B : PMIOPort  Port=1  Side=Left
  F : PMIOPort  Port=2  Side=Right
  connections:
  Transform3/RConn1 -- F/RConn1
  Solid/RConn1 -- Transform1/LConn1 -- ReferenceFrame/RConn1 -- Transform3/LConn1
  Transform1/RConn1 -- B/RConn1

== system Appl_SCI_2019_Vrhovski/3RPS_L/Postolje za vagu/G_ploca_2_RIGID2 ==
  ReferenceFrame : sm_lib/Frames and Transforms/Reference Frame  BlockFunction=simmechanics.library.frames_transforms.reference_frame
  Solid : sm_lib/Body Elements/Solid  InertiaType=Custom  Mass=5  MassUnits=kg  CenterOfMass=[-1.0925911726464245e-05 0 -4.4436244658035022]  CenterOfMassUnits=mm  MomentsOfInertia=[45540 79860 45540]  MomentsOfInertiaUnits=kg*mm^2  ProductsOfInertia=[0 -0.00010369999054466602 0]  ProductsOfInertiaUnits=kg*mm^2  DensityBased=on  Density=1000  DensityUnits=kg/(m^3)  GraphicType=FromGeometry  MarkerShape=Sphere  MarkerSize=10  MarkerSizeUnits=m  GraphicVisPropType=SimpleVisualProperties  GraphicDiffuseColor=[0.8 0.8 0.8]  GraphicSpecularColor=[0.5 0.5 0.5 1.0]  GraphicAmbientColor=[0.15 0.15 0.15 1.0]  GraphicEmissiveColor=[0.0 0.0 0.0 1.0]  GraphicShininess=75  GraphicOpacity=1  GeometryShape=Brick  RectangleSize=[1 1]  RectangleSizeUnits=m  BrickDimensions=[100 65 40]  BrickDimensionUnits=mm  CylinderRadius=120  CylinderRadiusUnits=mm  CylinderLength=20  CylinderLengthUnits=mm  SphereRadius=1  SphereRadiusUnits=m  EllipsoidRadii=[1 1 1]  EllipsoidRadiiUnits=m  ExtrusionCrossSection=[1 1; -1 1; -1 -1; 1 -1]  ExtrusionCrossSectionUnits=m  ExtrusionLength=1  ExtrusionLengthUnits=m  PolygonNumSides=3  PolygonOuterRadius=1  PolygonOuterRadiusUnits=m  ExtGeomFileType=STL  ExtGeomFileName=G_ploca_Default_sldprt.STL  ExtGeomFileUnits=mm  RevolutionCrossSection=[1 1; 1 -1; 2 -1; 2 1]  RevolutionCrossSectionUnits=m  RevolutionExtent=Full  RevolutionAngle=180  RevolutionAngleUnits=deg  BlockFunction=simmechanics.library.body_elements.solid
  Transform1 : sm_lib/Frames and Transforms/Rigid Transform  TranslationMethod=None  TranslationLengthUnit=mm  TranslationStandardAxis=-Z  TranslationStandardOffset=35.5  TranslationCartesianOffset="[-50.0000   86.6025         -10]"  TranslationROffset=0  TranslationROffsetUnits=m  TranslationZOffset=0  TranslationZOffsetUnits=m  TranslationThetaOffset=0  TranslationThetaOffsetUnits=deg  RotationMethod=ArbitraryAxis  RotationAngleUnits=rad  RotationStandardAxis=+Z  RotationAngle=0  RotationArbitraryAxis=[0 0 0]  FollAlignAxisA=+X  BaseAlignAxisA=+Y  FollAlignAxisB=+Y  BaseAlignAxisB=+Z  BlockFunction=simmechanics.library.frames_transforms.rigid_transform
  Transform3 : sm_lib/Frames and Transforms/Rigid Transform  TranslationMethod=None  TranslationLengthUnit=mm  TranslationStandardAxis=+Z  TranslationStandardOffset=35.5  TranslationCartesianOffset=[80.000000000002558 4.2632564145606011e-14 -32.999999999999048]  TranslationROffset=0  TranslationROffsetUnits=m  TranslationZOffset=0  TranslationZOffsetUnits=m  TranslationThetaOffset=0  TranslationThetaOffsetUnits=deg  RotationMethod=None  RotationAngleUnits=rad  RotationStandardAxis=+Z  RotationAngle=0  RotationArbitraryAxis=[0 0 0]  FollAlignAxisA=+X  BaseAlignAxisA=+Y  FollAlignAxisB=+Y  BaseAlignAxisB=+Z  BlockFunction=simmechanics.library.frames_transforms.rigid_transform
  B : PMIOPort  Port=1  Side=Left
  F : PMIOPort  Port=2  Side=Right
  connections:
  Transform1/RConn1 -- B/RConn1
  Transform1/LConn1 -- ReferenceFrame/RConn1 -- Solid/RConn1 -- Transform3/LConn1
  Transform3/RConn1 -- F/RConn1

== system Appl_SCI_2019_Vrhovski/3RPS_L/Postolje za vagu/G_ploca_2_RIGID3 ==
  ReferenceFrame : sm_lib/Frames and Transforms/Reference Frame  BlockFunction=simmechanics.library.frames_transforms.reference_frame
  Solid : sm_lib/Body Elements/Solid  InertiaType=Custom  Mass=5  MassUnits=kg  CenterOfMass=[-1.0925911726464245e-05 0 -4.4436244658035022]  CenterOfMassUnits=mm  MomentsOfInertia=[45540 79860 45540]  MomentsOfInertiaUnits=kg*mm^2  ProductsOfInertia=[0 -0.00010369999054466602 0]  ProductsOfInertiaUnits=kg*mm^2  DensityBased=on  Density=1000  DensityUnits=kg/(m^3)  GraphicType=FromGeometry  MarkerShape=Sphere  MarkerSize=10  MarkerSizeUnits=m  GraphicVisPropType=SimpleVisualProperties  GraphicDiffuseColor=[0.4 0.4 0.4]  GraphicSpecularColor=[0.5 0.5 0.5 1.0]  GraphicAmbientColor=[0.15 0.15 0.15 1.0]  GraphicEmissiveColor=[0.0 0.0 0.0 1.0]  GraphicShininess=75  GraphicOpacity=1  GeometryShape=Brick  RectangleSize=[1 1]  RectangleSizeUnits=m  BrickDimensions=[380 210 11]  BrickDimensionUnits=mm  CylinderRadius=120  CylinderRadiusUnits=mm  CylinderLength=20  CylinderLengthUnits=mm  SphereRadius=1  SphereRadiusUnits=m  EllipsoidRadii=[1 1 1]  EllipsoidRadiiUnits=m  ExtrusionCrossSection=[1 1; -1 1; -1 -1; 1 -1]  ExtrusionCrossSectionUnits=m  ExtrusionLength=1  ExtrusionLengthUnits=m  PolygonNumSides=3  PolygonOuterRadius=1  PolygonOuterRadiusUnits=m  ExtGeomFileType=STL  ExtGeomFileName=G_ploca_Default_sldprt.STL  ExtGeomFileUnits=mm  RevolutionCrossSection=[1 1; 1 -1; 2 -1; 2 1]  RevolutionCrossSectionUnits=m  RevolutionExtent=Full  RevolutionAngle=180  RevolutionAngleUnits=deg  BlockFunction=simmechanics.library.body_elements.solid
  Transform1 : sm_lib/Frames and Transforms/Rigid Transform  TranslationMethod=StandardAxis  TranslationLengthUnit=mm  TranslationStandardAxis=-Z  TranslationStandardOffset=25.5  TranslationCartesianOffset="[-50.0000   86.6025         -10]"  TranslationROffset=0  TranslationROffsetUnits=m  TranslationZOffset=0  TranslationZOffsetUnits=m  TranslationThetaOffset=0  TranslationThetaOffsetUnits=deg  RotationMethod=ArbitraryAxis  RotationAngleUnits=rad  RotationStandardAxis=+Z  RotationAngle=0  RotationArbitraryAxis=[0 0 0]  FollAlignAxisA=+X  BaseAlignAxisA=+Y  FollAlignAxisB=+Y  BaseAlignAxisB=+Z  BlockFunction=simmechanics.library.frames_transforms.rigid_transform
  Transform3 : sm_lib/Frames and Transforms/Rigid Transform  TranslationMethod=StandardAxis  TranslationLengthUnit=mm  TranslationStandardAxis=+Z  TranslationStandardOffset=5.5  TranslationCartesianOffset=[80.000000000002558 4.2632564145606011e-14 -32.999999999999048]  TranslationROffset=0  TranslationROffsetUnits=m  TranslationZOffset=0  TranslationZOffsetUnits=m  TranslationThetaOffset=0  TranslationThetaOffsetUnits=deg  RotationMethod=None  RotationAngleUnits=rad  RotationStandardAxis=+Z  RotationAngle=0  RotationArbitraryAxis=[0 0 0]  FollAlignAxisA=+X  BaseAlignAxisA=+Y  FollAlignAxisB=+Y  BaseAlignAxisB=+Z  BlockFunction=simmechanics.library.frames_transforms.rigid_transform
  B : PMIOPort  Port=1  Side=Left
  F : PMIOPort  Port=2  Side=Right
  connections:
  Transform3/RConn1 -- F/RConn1
  Transform1/RConn1 -- B/RConn1
  Solid/RConn1 -- Transform3/LConn1 -- Transform1/LConn1 -- ReferenceFrame/RConn1
